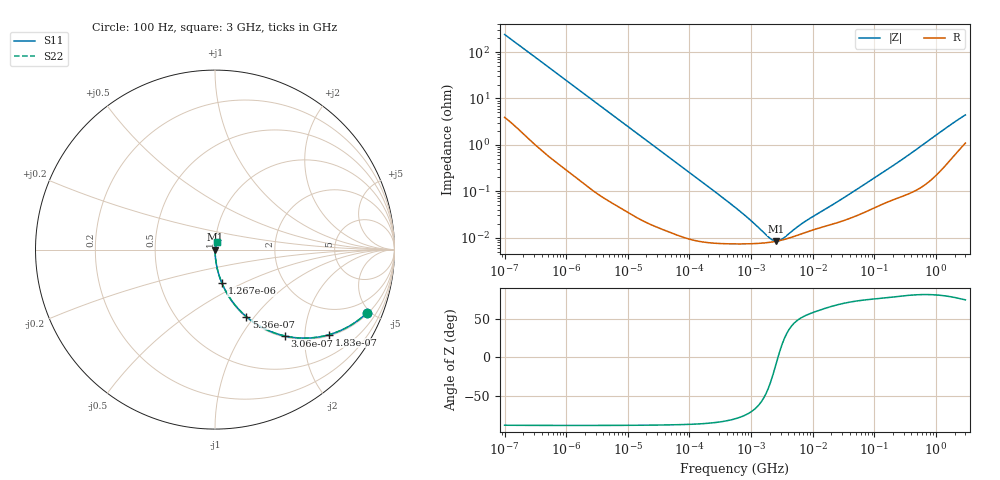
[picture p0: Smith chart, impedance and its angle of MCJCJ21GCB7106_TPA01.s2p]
! MCJCJ21GCB7106_TPA01  S-PARAMETER MODEL  ( Standard Model )
! Model Generated by TAIYO YUDEN Corporation (http://www.ty-top.com)
! Version 1.0
! TAIYO YUDEN Control No. 220601
! Copyright(c) 2015 TAIYO YUDEN CO.,LTD. All Rights Reserved.
! Product Description (link to TY-COMPAS)
! https://ds.yuden.co.jp/TYCOMPAS/or/detail?pn=MCJCJ21GCB7106KTPA01&u=M
! Products Name : Multilayer Ceramic Capacitors
! Characteristics :
!  Capacitance : 10 [uF] , Rated Voltage : 6.3 [V] , TCC : X7R
!  Case Size : 2.0 x 1.25 / 0.079 x 0.049 [mm/inch] , Thickness : 1.25 / 0.049 [mm/inch]
!  (Conditions: Temperature = 25 [degC] , DC Bias Voltage = 0 [V])
! External Node Assignments :
!  1  o---| |---o  2
! GND o---------o GND
! Frequency Range : 100Hz  -  3GHz  [ 401 STEP ]
# MHZ S RI R 50
! Freq[MHz].  S11 Real  S11 Imag  S21 Real  S21 Imag  S12 Real  S12 Imag  S22 Real  S22 Imag
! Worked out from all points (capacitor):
!   401 points, 100 Hz to 3 GHz, reference 50 ohm
!   read as one part in series: C = 6.61 uF near 109 Hz
!   lowest |Z| = 8.38 mohm at 2.579 MHz (marker M1)
!   series resonance near 2.723 MHz, so ESL is about 520 pH
!   S11 on the Smith chart (normalised r, x): 100 Hz: 1.08, -4.80; 183 Hz: 1.04, -2.65; 306 Hz: 1.02, -1.59; 536 Hz: 1.01, -0.91; 1.267 kHz: 1.00, -0.39; 3 GHz: 1.02, +0.09
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0.0001  0.8481 -0.3508  0.1519 0.3508  0.1519 0.3508  0.8481 -0.3508
0.000124  0.7867 -0.4018  0.2133 0.4018  0.2133 0.4018  0.7867 -0.4018
0.000183  0.6349 -0.4742  0.3651 0.4742  0.3651 0.4742  0.6349 -0.4742
0.000306  0.3878 -0.4808  0.6122 0.4808  0.6122 0.4808  0.3878 -0.4808
0.000536  0.1746 -0.3737  0.8254 0.3737  0.8254 0.3737  0.1746 -0.3737
0.000789  0.0903 -0.2808  0.9097 0.2808  0.9097 0.2808  0.0903 -0.2808
0.001267  0.0381 -0.1858  0.9619 0.1858  0.9619 0.1858  0.0381 -0.1858
0.001788  0.02 -0.1346  0.98 0.1346  0.98 0.1346  0.02 -0.1346
0.005476  0.0026 -0.0451  0.9974 0.0451  0.9974 0.0451  0.0026 -0.0451
0.031977  0.000222 -0.00784  0.9998 0.00784  0.9998 0.00784  0.000222 -0.00784
0.547723  7.31e-05 -0.000444  0.9999 0.000444  0.9999 0.000444  7.31e-05 -0.000444
1.000599  7.36e-05 -0.000218  0.9999 0.000218  0.9999 0.000218  7.36e-05 -0.000218
1.827928  7.77e-05 -7.48e-05  0.9999 7.48e-05  0.9999 7.48e-05  7.77e-05 -7.48e-05
2.079876  7.94e-05 -4.95e-05  0.9999 4.95e-05  0.9999 4.95e-05  7.94e-05 -4.95e-05
2.579298  8.32e-05 -9.69e-06  0.9999 9.69e-06  0.9999 9.69e-06  8.32e-05 -9.69e-06
3.639519  9.28e-05 5.1e-05  0.9999 -5.1e-05  0.9999 -5.1e-05  9.28e-05 5.1e-05
6.10039  0.000116 0.000143  0.9999 -0.000143  0.9999 -0.000143  0.000116 0.000143
9.794414  0.000144 0.000238  0.9999 -0.000238  0.9999 -0.000238  0.000144 0.000238
29.99103  0.000226 0.000647  0.9998 -0.000647  0.9998 -0.000647  0.000226 0.000647
175.1444  0.000614 0.00309  0.9994 -0.00309  0.9994 -0.00309  0.000614 0.00309
1714.41  0.00539 0.0262  0.9946 -0.0262  0.9946 -0.0262  0.00539 0.0262
3000  0.0125 0.0418  0.9875 -0.0418  0.9875 -0.0418  0.0125 0.0418
